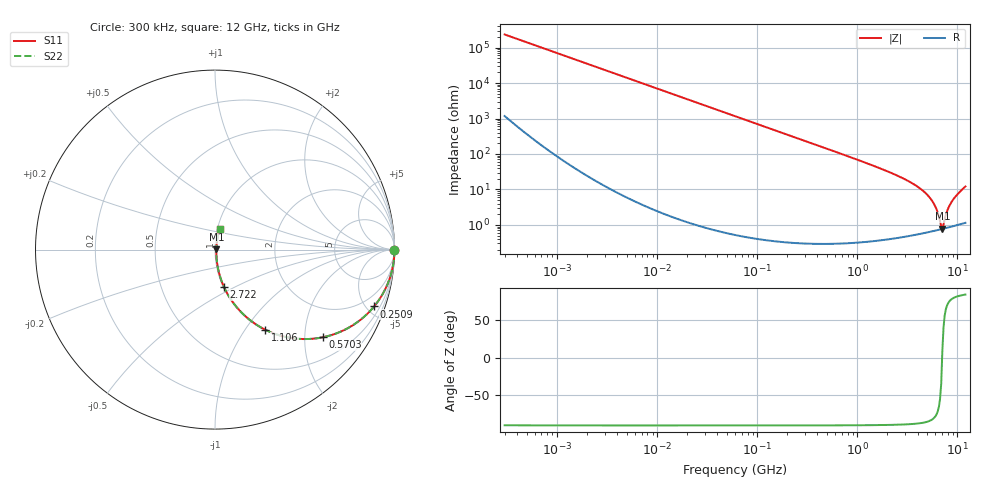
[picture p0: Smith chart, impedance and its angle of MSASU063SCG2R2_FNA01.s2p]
! MSASU063SCG2R2_FNA01  S-PARAMETER MODEL  ( Standard Model )
! Model Generated by TAIYO YUDEN Corporation (http://www.ty-top.com)
! Version 1.0
! TAIYO YUDEN Control No. 240819
! Copyright(c) 2024 TAIYO YUDEN CO.,LTD. All Rights Reserved.
! Product Description (link to TY-COMPAS)
! https://ds.yuden.co.jp/TYCOMPAS/or/detail?pn=MSASU063SCG2R2CFNA01&u=M
! Products Name : Multilayer Ceramic Capacitors
! Characteristics :
!  Capacitance : 2.2 [pF] , Rated Voltage : 50 [V] , TCC : CG / C0G
!  Case Size : 0.6 x 0.3 / 0.024 x 0.012 [mm/inch] , Thickness : 0.3 / 0.012 [mm/inch]
!  (Conditions: Temperature = 25 [degC] , DC Bias Voltage = 0 [V])
! External Node Assignments :
!  1  o---| |---o  2
! GND o---------o GND
! Frequency Range : 0.3MHz  -  12000MHz  [ 401 STEP ]
# MHZ S RI R 50
! Freq[MHz].  S11 Real  S11 Imag  S21 Real  S21 Imag  S12 Real  S12 Imag  S22 Real  S22 Imag
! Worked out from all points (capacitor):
!   401 points, 300 kHz to 12 GHz, reference 50 ohm
!   read as one part in series: C = 2.26 pF near 316.3 kHz
!   lowest |Z| = 778 mohm at 7.064 GHz (marker M1)
!   series resonance near 7.029 GHz, so ESL is about 230 pH
!   S11 on the Smith chart (normalised r, x): 300 kHz: open; 250.9 MHz: 1.01, -5.60; 570.3 MHz: 1.01, -2.45; 1.106 GHz: 1.01, -1.24; 2.722 GHz: 1.01, -0.44; 12 GHz: 1.02, +0.24
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0.3  1 -0.000427  2.32e-06 0.000427  2.32e-06 0.000427  1 -0.000427
1.769972  1 -0.00252  8.23e-06 0.00252  8.23e-06 0.00252  1 -0.00252
10.44266  0.9998 -0.0149  0.000226 0.0149  0.000226 0.0149  0.9998 -0.0149
60  0.9927 -0.0848  0.00727 0.0848  0.00727 0.0848  0.9927 -0.0848
140.0606  0.9616 -0.1917  0.0384 0.1917  0.0384 0.1917  0.9616 -0.1917
250.8588  0.8865 -0.3167  0.1135 0.3167  0.1135 0.3167  0.8865 -0.3167
353.9943  0.7965 -0.4019  0.2035 0.4019  0.2035 0.4019  0.7965 -0.4019
570.2811  0.5996 -0.4888  0.4004 0.4888  0.4004 0.4888  0.5996 -0.4888
1105.905  0.2786 -0.4457  0.7214 0.4457  0.7214 0.4457  0.2786 -0.4457
2088.533  0.0891 -0.2786  0.9109 0.2786  0.9109 0.2786  0.0891 -0.2786
2722.03  0.0499 -0.2079  0.9501 0.2079  0.9501 0.2079  0.0499 -0.2079
3944.255  0.0199 -0.1195  0.9801 0.1195  0.9801 0.1195  0.0199 -0.1195
5140.631  0.0102 -0.0632  0.9898 0.0632  0.9898 0.0632  0.0102 -0.0632
5868.704  0.00807 -0.0364  0.9919 0.0364  0.9919 0.0364  0.00807 -0.0364
6188.031  0.00765 -0.0259  0.9924 0.0259  0.9924 0.0259  0.00765 -0.0259
6699.894  0.00746 -0.0102  0.9925 0.0102  0.9925 0.0102  0.00746 -0.0102
7064.448  0.00762 0.00123  0.9924 -0.00123  0.9924 -0.00123  0.00762 0.00123
7254.098  0.0078 0.00655  0.9922 -0.00655  0.9922 -0.00655  0.0078 0.00655
8064.993  0.0091 0.0271  0.9909 -0.0271  0.9909 -0.0271  0.0091 0.0271
8732.115  0.0107 0.0427  0.9893 -0.0427  0.9893 -0.0427  0.0107 0.0427
9968.853  0.0147 0.0696  0.9853 -0.0696  0.9853 -0.0696  0.0147 0.0696
12000  0.0252 0.1163  0.9748 -0.1163  0.9748 -0.1163  0.0252 0.1163
